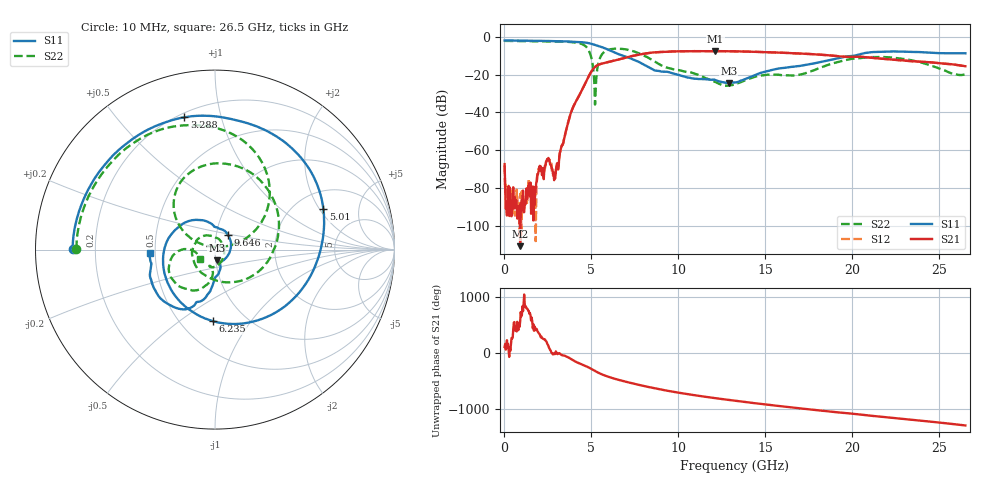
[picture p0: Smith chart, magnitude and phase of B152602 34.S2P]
!  2-Port S-parameters saved by WinCal
! VAR MeasName=S-Parameters (CALIBRATED_DATA) read from VNA (N5242A)
! VAR MeasDate=2016-1-5 16:31:15
! VAR NAME=B152602 34
! VAR FILENAME=B152602 34.S2P
! VAR DATE=2016-1-5 16:31:15
! VAR PHYS_PORTS=1,2
# Hz S DB R 50
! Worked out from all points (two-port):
!   801 points, 10 MHz to 26.5 GHz, reference 50 ohm
!   highest |S21| = -7.63 dB at 12.13 GHz (marker M1); lowest = -110.5 dB at 904 MHz (marker M2)
!   |S21| within 3 dB of the highest: 7.158 GHz to 19.57 GHz (12.41 GHz wide, 92.9 % of centre); 19.88 GHz to 20.54 GHz (661.4 MHz wide, 3.27 % of centre)
!   lowest |S11| = -24.4 dB at 12.89 GHz (marker M3), VSWR 1.13, Z = 50.6 - j6.07 ohm
!   |S11| at or under -10 dB: 6.788 GHz to 20.15 GHz (13.36 GHz wide, 99.2 % of centre)
!   |S22| runs from -35.8 to -2.2 dB; largest |S21 - S12| = 0.0032
!   S11 on the Smith chart (normalised r, x): 10 MHz: 0.12, +0.00; 3.288 GHz: 0.22, +0.77; 5.01 GHz: 2.81, +2.17; 6.235 GHz: 0.71, -0.68; 9.646 GHz: 1.14, +0.19; 26.5 GHz: 0.47, -0.02
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1e7  -2.01 179.8  -67.23 110.3  -67.92 85.1  -2.24 179.8
1.755625e8  -2.02 176.4  -86.96 148.8  -87.24 52.5  -2.24 177.3
9.040375e8  -2.10 161.4  -110.52 -157.2  -82.95 140.0  -2.28 166.0
1.698738e9  -2.20 144.7  -79.35 39.4  -84.89 98.3  -2.36 153.3
2.460325e9  -2.28 126.8  -64.54 167.0  -64.65 167.7  -2.44 139.9
2.857675e9  -2.34 116.2  -75.74 -13.3  -74.10 -35.9  -2.48 131.9
3.288138e9  -2.42 103.1  -57.53 -32.2  -57.62 -32.5  -2.58 121.9
4.447075e9  -2.94 56.2  -28.40 156.7  -28.38 156.8  -3.88 78.6
5.009988e9  -3.81 20.5  -18.22 73.5  -18.23 73.6  -11.69 26.6
5.241775e9  -4.47 3.7  -15.74 32.2  -15.73 32.4  -28.72 149.7
5.5729e9  -5.45 -23.6  -14.29 -18.5  -14.29 -18.4  -9.81 135.2
6.23515e9  -7.97 -91.4  -12.79 -91.6  -12.77 -91.4  -6.45 94.3
7.526538e9  -12.54 146.2  -9.88 163.7  -9.86 163.7  -8.05 26.4
8.851038e9  -18.09 86.9  -8.16 74.2  -8.16 74.1  -14.34 -71.7
9.645738e9  -19.26 47.6  -7.81 28.7  -7.82 28.7  -17.02 -139.5
1.212918e10  -22.95 -77.8  -7.63 -89.0  -7.65 -89.0  -23.93 72.9
1.289076e10  -24.37 -81.2  -7.73 -121.0  -7.72 -120.8  -25.81 9.0
1.3255e10  -24.20 -77.9  -7.75 -135.3  -7.74 -135.3  -25.13 -23.2
1.494374e10  -18.55 -76.6  -8.18 160.4  -8.16 160.2  -20.27 -93.5
1.769208e10  -14.27 -93.4  -9.23 64.2  -9.20 64.4  -18.08 -95.4
2.209604e10  -7.80 -137.7  -11.96 -75.9  -11.90 -76.4  -10.91 -153.4
2.65e10  -8.78 -177.0  -15.60 141.6  -15.62 141.4  -19.95 -147.5
